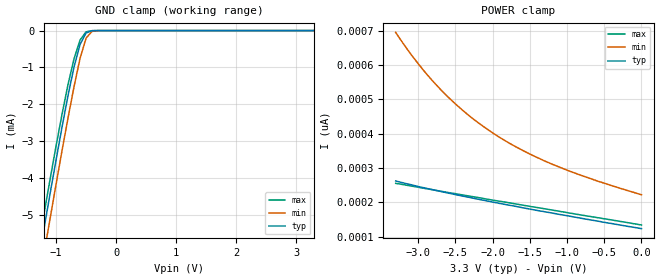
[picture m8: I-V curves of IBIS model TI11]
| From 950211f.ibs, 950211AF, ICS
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|   Model TI11
[Model]   TI11
Model_type   Input
Polarity   Non-Inverting
Vinl = 800.00mV
Vinh =   2.00V
C_comp   5.50pF   5.00pF   6.00pF
[Temperature Range]   27.00   70.00   0.00
[Voltage Range]   3.30V   3.00V   3.70V
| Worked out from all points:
|   GND clamp passes 1 mA (typ) near -0.70 V on its own axis
[GND_clamp]
| voltage   I(typ)   I(min)   I(max)
-3.3V     -25.94mA   -26.62mA   -25.53mA
-1.3V     -6.33mA    -7.02mA    -5.92mA
-1.2V     -5.38mA    -6.06mA    -4.98mA
-1.1V     -4.44mA    -5.12mA    -4.05mA
-900mV    -2.62mA    -3.26mA    -2.27mA
-800mV    -1.76mA    -2.37mA    -1.46mA
-700mV    -985.4uA   -1.52mA    -763uA
-600mV    -374.8uA   -752.5uA   -256.1uA
-500mV    -64.68uA   -205.4uA   -34.13uA
-400mV    -4.39uA    -20.4uA    -1.64uA
-300mV    -160.8nA   -1.11uA    -40.61nA
3.3V      123pA      241.6pA    119.2pA
[POWER_clamp]
| voltage   I(typ)   I(min)   I(max)
-3.3V     261.8pA    694.5pA    254.9pA
-3.1V     251.2pA    632.1pA    247.4pA
-3V       245.8pA    604pA      243.7pA
-2.9V     241pA      577.1pA    239.7pA
-2.7V     231.5pA    528.9pA    232.3pA
-2.4V     217.8pA    467.4pA    221.1pA
-2.2V     209pA      432.6pA    213.9pA
-2V       200.6pA    402.1pA    206.2pA
-1.6V     184.1pA    351.4pA    191.7pA
-1.2V     168.5pA    310.8pA    177.2pA
-600mV    145.5pA    262.3pA    155.4pA
0V        123pA      221.7pA    133.7pA
